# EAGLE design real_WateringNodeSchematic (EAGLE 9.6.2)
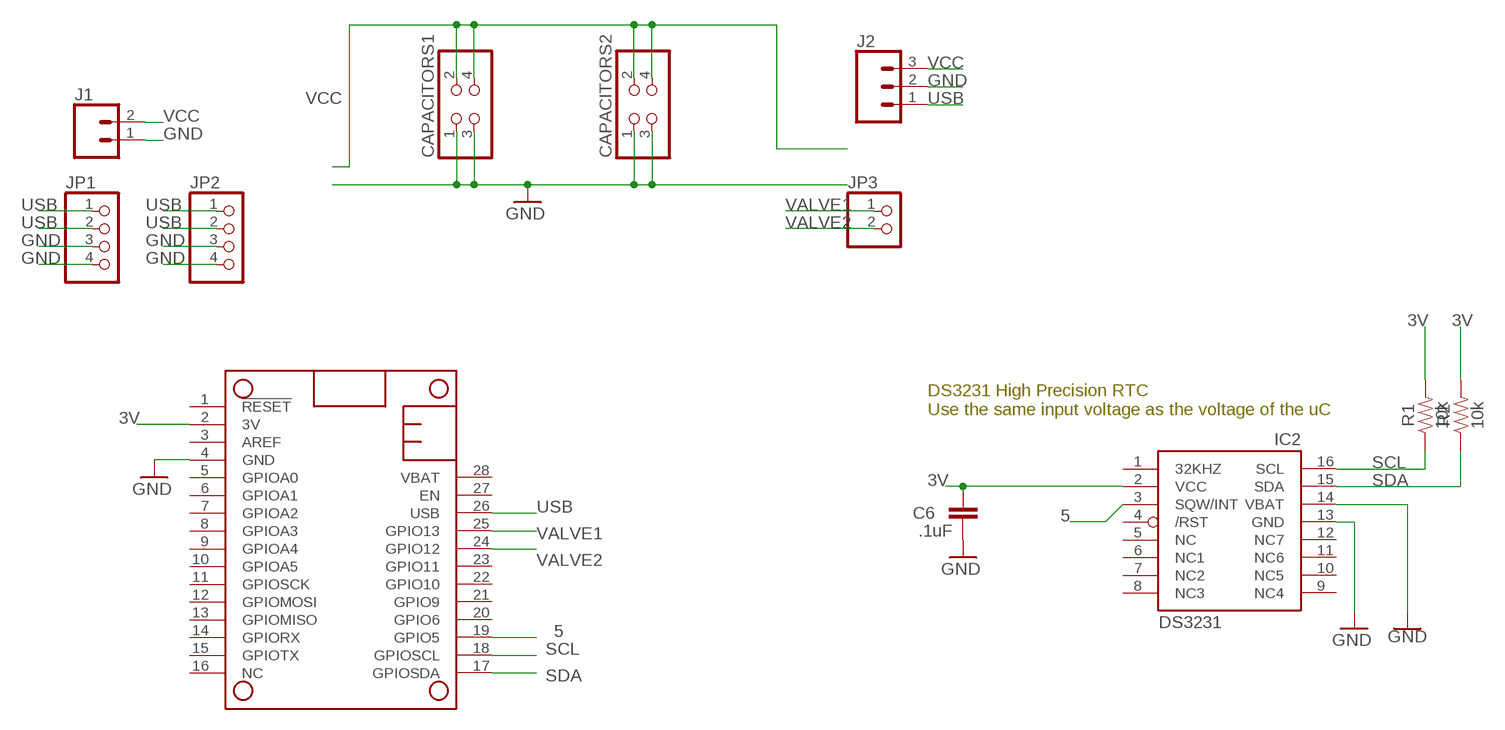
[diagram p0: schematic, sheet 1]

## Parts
C6  .1uF  CC1206  [C1206]
CAPACITORS1  PINHD-2X2  [2X02]
CAPACITORS2  PINHD-2X2  [2X02]
IC2  DS3231/SO  [SO16W]
J1  CONN_023.5MM_LOCK  [SCREWTERMINAL-3.5MM-2_LOCK]
J2  CONN_03SCREW  [SCREWTERMINAL-3.5MM-3]
JP1  PINHD-1X4  [1X04]
JP2  PINHD-1X4  [1X04]
JP3  PINHD-1X2  [1X02]
MS1  FEATHERWING_NODIM  [FEATHERWING_DIM]
R1  10k  0.27OHM-0603-1/10W-1%  [0603]
R2  10k  0.27OHM-0603-1/10W-1%  [0603]

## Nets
3V: C6.1 IC2.2(VCC) MS1.2(3V) R1.2 R2.2
5: IC2.3(SQW/INT) MS1.19(GPIO5)
GND: C6.2 CAPACITORS1.1 CAPACITORS1.3 CAPACITORS2.1 CAPACITORS2.3 IC2.13(GND) IC2.14(VBAT) J1.1 J2.2 JP1.3 JP1.4 JP2.3 JP2.4 MS1.4(GND)
SCL: IC2.16(SCL) MS1.18(GPIOSCL) R1.1
SDA: IC2.15(SDA) MS1.17(GPIOSDA) R2.1
USB: J2.1 JP1.1 JP1.2 JP2.1 JP2.2 MS1.26(USB)
VALVE1: JP3.1 MS1.25(GPIO13)
VALVE2: JP3.2 MS1.24(GPIO12)
VCC: CAPACITORS1.2 CAPACITORS1.4 CAPACITORS2.2 CAPACITORS2.4 J1.2 J2.3
Unconnected: IC2.1(32KHZ) IC2.4(/RST) IC2.5(NC) IC2.6(NC1) IC2.7(NC2) IC2.8(NC3) IC2.9(NC4) IC2.10(NC5) IC2.11(NC6) IC2.12(NC7) MS1.1(!RESET) MS1.3(AREF) MS1.5(GPIOA0) MS1.6(GPIOA1) MS1.7(GPIOA2) MS1.8(GPIOA3) MS1.9(GPIOA4) MS1.10(GPIOA5) MS1.11(GPIOSCK) MS1.12(GPIOMOSI) MS1.13(GPIOMISO) MS1.14(GPIORX) MS1.15(GPIOTX) MS1.16(NC) MS1.20(GPIO6) MS1.21(GPIO9) MS1.22(GPIO10) MS1.23(GPIO11) MS1.27(EN) MS1.28(VBAT)

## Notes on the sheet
- DS3231 High Precision RTC
  Use the same input voltage as the voltage of the uC

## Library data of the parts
C6 = eagle-ltspice:C: CAPACITOR, European symbol; SPICEMODEL: NONE; SPICEPREFIX: C
CAPACITORS1 CAPACITORS2 = pinhead:PINHD-2X2: PIN HEADER
IC2 = adafruit:DS3231
J1 = SparkFun-Connectors:CONN_02: Multi connection point. Often used as Generic Header-pin footprint for 0.1 inch spaced/style header connections; PROD_ID: CONN-08399
J2 = SparkFun-Connectors:CONN_03: Multi connection point. Often used as Generic Header-pin footprint for 0.1 inch spaced/style header connections On any of the 0.1 inch spaced packages, you can populate with these: Break Away Headers - Straight (PRT-00116) Break Away Male Headers - Right Angle (PRT-00553) Female Headers (PRT-00115)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; PROD_ID: CONN-08288; SF_ID: PRT-08235
JP1 JP2 = pinhead:PINHD-1X4: PIN HEADER
JP3 = pinhead:PINHD-1X2: PIN HEADER
MS1 = adafruit:FEATHERWING
R1 R2 = SparkFun-Resistors:0.27OHM: 0.27Ω resistor; PROD_ID: RES-08787; VALUE: 0.27

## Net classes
0 default: width 0.203 mm, drill 0.203 mm, clearance 0.178 mm
2 Power2: width 0.457 mm, drill 0.457 mm, clearance 0.178 mm

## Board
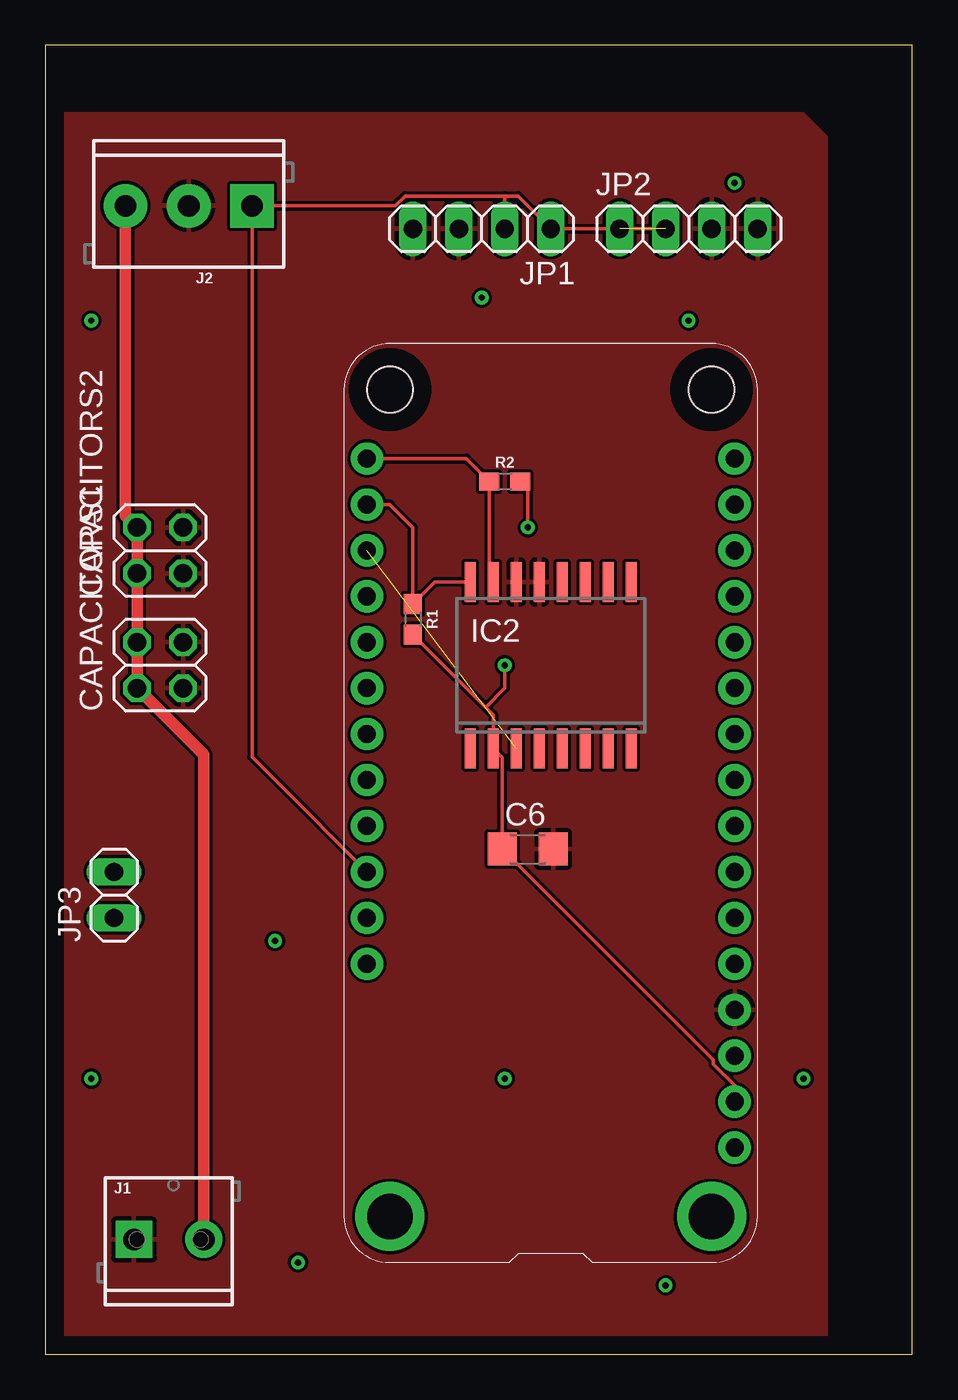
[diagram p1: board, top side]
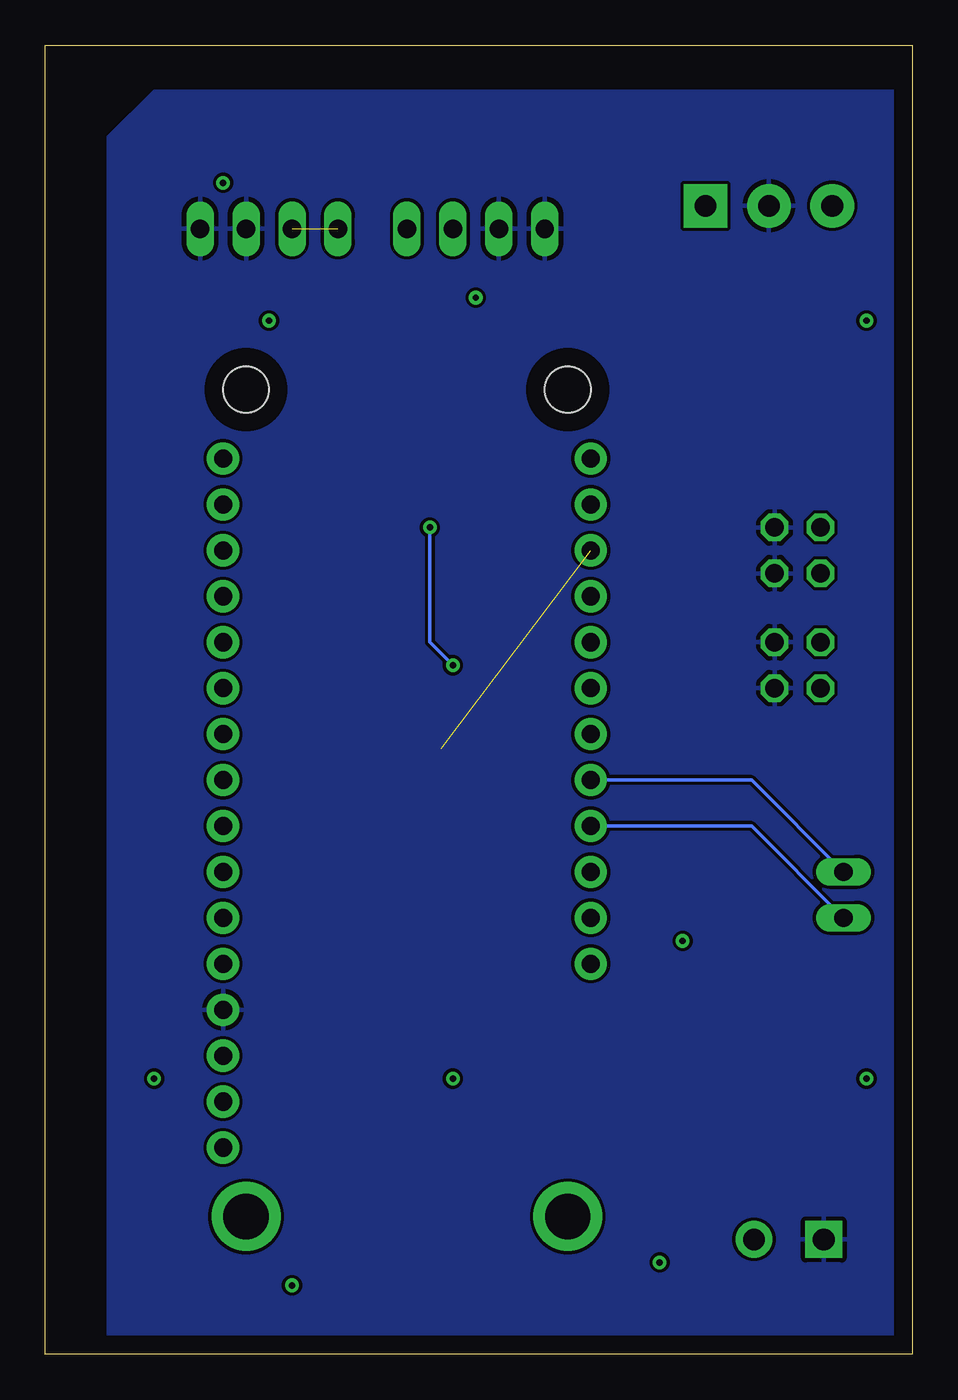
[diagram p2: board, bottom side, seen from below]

Size 47.93 x 72.38 mm. Coordinates in mm from the lower left corner, seen from the top.
Outline: 0,0 47.93,0 47.93,72.38 0,72.38 0,0
Copper layers (1*16): Top 0.035mm / dielectric 1.5mm / Bottom 0.035mm
Design rules "default": minimum track width 6mil, minimum drill 0.35mm, track to track 6mil, track to pad 6mil, pad to pad 6mil, via to via 6mil, smd to smd 6mil, copper to edge 40mil, drill to drill 6mil, minimum pad ring 10mil, minimum via ring 8mil, stop-mask expansion 4mil, vias tented up to drill 0mil, thermal gap 10mil

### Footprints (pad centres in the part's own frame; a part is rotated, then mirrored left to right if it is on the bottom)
C1206 = smd 1.6 x 1.8: 1 -1.4,0; 2 1.4,0
2X02 = drill 1.016 octagon: 1 -1.27,-1.27; 2 -1.27,1.27; 3 1.27,-1.27; 4 1.27,1.27
SO16W = smd 0.6 x 2.2: 1 -4.445,-4.6; 2 -3.175,-4.6; 3 -1.905,-4.6; 4 -0.635,-4.6; 5 0.635,-4.6; 6 1.905,-4.6; 7 3.175,-4.6; 8 4.445,-4.6; 9 4.445,4.6; 10 3.175,4.6; 11 1.905,4.6; 12 0.635,4.6; 13 -0.635,4.6; 14 -1.905,4.6; 15 -3.175,4.6; 16 -4.445,4.6
SCREWTERMINAL-3.5MM-2_LOCK = drill 1.2 pad 2.032 square: 1 -0.178,0 | drill 1.2 pad 2.032: 2 3.678,0
SCREWTERMINAL-3.5MM-3 = drill 1.2 pad 2.413 square: 1 0,0 | drill 1.2 pad 2.413: 2 3.5,0; 3 7,0
1X04 = drill 1.016 long: 1 -3.81,0; 2 -1.27,0; 3 1.27,0; 4 3.81,0
1X02 = drill 1.016 long: 1 -1.27,0; 2 1.27,0
FEATHERWING_DIM = drill 1 pad 1.778: 1 6.35,1.27; 2 8.89,1.27; 3 11.43,1.27; 4 13.97,1.27; 5 16.51,1.27; 6 19.05,1.27; 7 21.59,1.27; 8 24.13,1.27; 9 26.67,1.27; 10 29.21,1.27; 11 31.75,1.27; 12 34.29,1.27; 13 36.83,1.27; 14 39.37,1.27; 15 41.91,1.27; 16 44.45,1.27; 17 44.45,21.59; 18 41.91,21.59; 19 39.37,21.59; 20 36.83,21.59; 21 34.29,21.59; 22 31.75,21.59; 23 29.21,21.59; 24 26.67,21.59; 25 24.13,21.59; 26 21.59,21.59; 27 19.05,21.59; 28 16.51,21.59 | drill 2.5 pad 3.81: P$1 2.54,20.32; P$2 2.54,2.54 | hole 2.54: 48.26,20.32; 48.26,2.54
0603 = smd 1.1 x 1: 1 -0.85,0; 2 0.85,0

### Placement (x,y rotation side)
C6  26.67,27.94 0 top
CAPACITORS1  6.35,38.1 90 top
CAPACITORS2  6.35,44.45 90 top
IC2  27.94,38.1 0 top
J1  5.08,6.35 0 top
J2  11.43,63.5 180 top
JP1  24.13,62.23 180 top
JP2  35.56,62.23 0 top
JP3  3.81,25.4 90 top
MS1  39.37,5.08 90 top
R1  20.32,40.64 270 top
R2  25.4,48.26 0 top

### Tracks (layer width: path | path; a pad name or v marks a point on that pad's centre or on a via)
3V  (via drill 0.35)
  Top 0.203: R1.2 24.34,35.77 | 24.34,35.77 24.77,35.34 IC2.2 25.27,32.99 C6.1 36.93,16.28 36.93,16.03 38.1,14.86 MS1.2 | R2.2 26.67,47.84 v26.67,45.72 | v25.4,38.1 25.4,36.83 24.34,35.77
  Bottom 0.203: v26.67,45.72 26.67,39.37 v25.4,38.1
5  (1 unrouted)
GND
  pour Top: 0,68.58 41.91,68.58 43.18,67.31 43.18,0 0,0
  pour Bottom: 0,69.85 41.91,69.85 44.45,67.31 44.45,-1.27 43.18,-2.54 1.27,-2.54 -1.27,0 -1.27,68.58
N$1  (via drill 0.35)
  other vias: 13.97,5.08
N$2  (via drill 0.35)
  other vias: 2.54,15.24
N$3  (via drill 0.35)
  other vias: 34.29,3.81
N$4  (via drill 0.35)
  other vias: 41.91,15.24
N$5  (via drill 0.35)
  other vias: 25.4,15.24
N$6  (via drill 0.35)
  other vias: 38.1,64.77
N$7  (via drill 0.35)
  other vias: 24.13,58.42
N$8  (via drill 0.35)
  other vias: 35.56,57.15
N$9  (via drill 0.35)
  other vias: 2.54,57.15
N$10  (via drill 0.35)
  other vias: 12.7,22.86
SCL
  Top 0.203: IC2.16 21.53,42.7 R1.1 20.32,45.72 19.05,46.99 MS1.18
SDA
  Top 0.203: MS1.17 23.28,49.53 R2.1 24.55,42.91 IC2.15
USB  (1 unrouted)
  Top 0.203: MS1.26 12.7,31.75 11.43,33.02 J2.1 19.36,63.5 19.89,64.03 25.4,64.03 | JP2.2 JP1.1 26.14,64.03 25.4,64.03 | JP1.2 25.4,64.03
VALVE1
  Bottom 0.203: JP3.1 8.89,29.21 MS1.25
VALVE2
  Bottom 0.203: JP3.2 8.89,31.75 MS1.24
VCC
  Top 0.203: CAPACITORS1.4 CAPACITORS2.2 CAPACITORS2.4
  Top 0.635: J1.2 8.76,33.15 CAPACITORS1.2 CAPACITORS1.4 CAPACITORS2.4 4.43,46.37 J2.3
